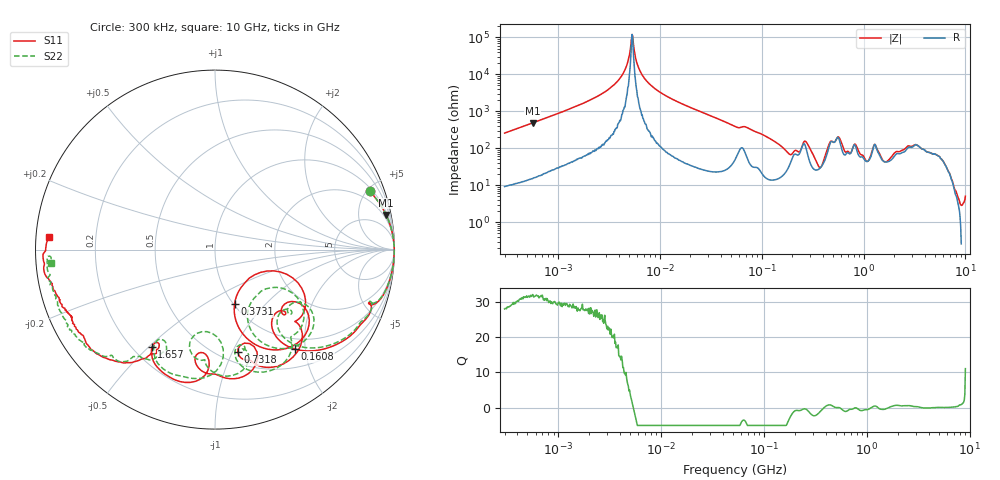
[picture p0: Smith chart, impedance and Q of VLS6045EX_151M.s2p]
! S-Parameter Data Generated by TDK Corporation
! Copyright(C) 2019 TDK Corporation.
! All Rights Reserved.
! TDK P/N: VLS6045EX-151M (Inductor)
! Property: L=150uH at 100kHz
! Size(LxWxT): 6x6x4.5mm
! Model Type: s2p (Touchstone File Format Version 1.0)
! Frequency: DC=Yes Start=0.3MHz Stop=10000MHz 802points Log-sweep
! Model Generated on May 10, 2019
! Port Assignments:
!  1 ---@@@--- 2
! Applicable Conditions:
!  Temperature = 25 degC
!  DC Bias Current = 0 A
!  Small Signal Operation
! Terms and conditions regarding TDK Simulation Models
! (1)This simulation model is being provided solely for informational purposes. Please refer to the specifications of the products in terms of detailed characteristics of such products.
! (2)In no event shall TDK Corporation of any of its subsidiaries be liable for any loss or damage arising, directly or indirectly,
!  From any information contained in this simulation model, including, but not limited to loss or damages arising from any inaccuracies, omissions or errors in connection with such information.
! (3)Any and all copyrights on this simulation model are owned by TDK Corporation.
!  Duplication or redistribution of this simulation model without prior written permission from TDK Corporation is prohibited.
! (4)This simulation model is subject to any modification or change without any prior notice.
! (5)Neither TDK Corporation nor any of its subsidiaries shall make any warranty, express or implied,
!  Including but not limited to the correctness, implied warranties of merchantability and fitness for a particular purpose with respect to this simulation models.
! (6)The use of this simulation model shall be deemed to have consented to the terms and conditions hereof.
# Hz S MA R 50
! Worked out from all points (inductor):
!   801 points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, 300 kHz to 10 GHz, reference 50 ohm
!   read as one part in series: L = 136 uH near 318.3 kHz
!   highest Q = 31.7 at 567.7 kHz (marker M1), where L = 137 uH
!   self-resonance near 5.354 MHz
!   S11 on the Smith chart (normalised r, x): 300 kHz: 1.21, +5.19; 160.8 MHz: 0.80, -1.80; 373.1 MHz: 1.01, -0.69; 731.8 MHz: 0.60, -1.05; 1.657 GHz: 0.27, -0.51; 10 GHz: 0.04, +0.04
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300000  0.9206 20.7  0.3574 -67.2  0.3576 -67.2  0.9207 20.7
567737  0.973 11.4  0.1994 -76.8  0.1995 -76.8  0.9731 11.4
1713600  0.9958 3.4  0.06289 -84.6  0.06291 -84.5  0.9959 3.4
3866967  0.9988 0.5  0.01512 -85.6  0.01513 -85.8  0.999 0.5
4611084  0.9991 -0.0  0.006961 -83.2  0.006975 -82.9  0.9992 0.0
5354396  0.9991 -0.5  0.0008341 -3.4  0.000786 -5.8  0.9993 -0.4
6556275  0.999 -1.1  0.009214 83.7  0.009301 84.0  0.9992 -1.1
9671944  0.9985 -2.5  0.02832 85.4  0.02833 85.5  0.9987 -2.4
5.477226e7  0.9411 -18.7  0.2394 64.4  0.2395 64.4  0.942 -18.2
1.608169e8  0.7105 -51.2  0.5997 31.0  0.5997 31.0  0.7147 -48.9
2.444933e8  0.5153 -34.1  0.4969 -7.3  0.4969 -7.3  0.5421 -32.6
3.126428e8  0.6129 -63.7  0.6067 9.9  0.6068 9.9  0.6333 -59.4
3.730642e8  0.3235 -70.4  0.7325 -15.4  0.7326 -15.4  0.3886 -61.8
4.74732e8  0.5932 -31.8  0.376 -43.5  0.376 -43.5  0.639 -40.0
5.99416e8  0.7421 -58.9  0.3375 -12.8  0.3376 -12.8  0.734 -68.4
7.318083e8  0.5853 -77.5  0.4709 -32.7  0.4711 -32.7  0.5813 -75.0
1.149233e9  0.5788 -97.9  0.496 -64.7  0.4968 -64.7  0.4636 -99.1
1.339606e9  0.7606 -104.7  0.2797 -60.3  0.2804 -60.3  0.7284 -99.8
1.657186e9  0.6483 -122.8  0.3998 -74.8  0.4016 -75.0  0.6397 -122.2
1.767019e9  0.6139 -122.5  0.3941 -87.0  0.396 -87.3  0.5936 -122.2
3.34571e9  0.8873 -141.3  0.0901 -123.3  0.08887 -123.1  0.8645 -137.3
1e10  0.9294 175.7  0.05035 -151.2  0.0506 -151.2  0.9187 -175.3
